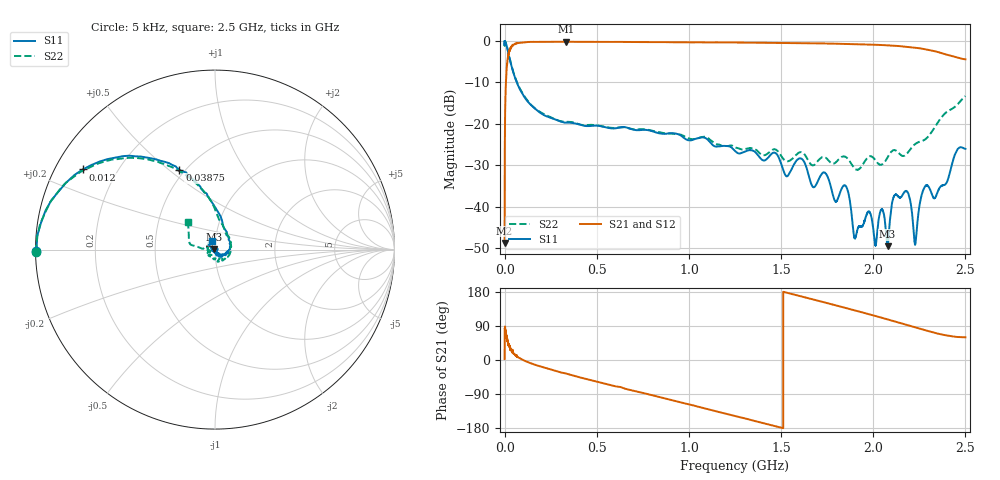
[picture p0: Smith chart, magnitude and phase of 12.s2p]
#  HZ  S  MA  R  50.00
! Rohde & Schwarz Vector Network Analyzer
! Rohde-Schwarz,ZNL6-2Port,1323001206101378,1.50.1.34-21.10.1.104
! Created: UTC 3/3/2025, 4:59:50 AM
! freq[Hz]  mag:S11  ang:S11  mag:S21  ang:S21  mag:S12  ang:S12  mag:S22  ang:S22
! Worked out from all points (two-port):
!   10001 points, 5 kHz to 2.5 GHz, reference 50 ohm
!   highest |S21| = -0.17 dB at 332 MHz (marker M1); lowest = -48.8 dB at 5 kHz (marker M2)
!   |S21| within 3 dB of the highest: 21.47 MHz to 2.389 GHz (2.367 GHz wide, 196 % of centre)
!   lowest |S11| = -49.5 dB at 2.078 GHz (marker M3), VSWR 1.01, Z = 49.7 + j0.0807 ohm
!   |S11| at or under -10 dB: 66.27 MHz to end of sweep
!   |S22| runs from -31.1 to 0.1 dB; largest |S21 - S12| = 0.17
!   S11 on the Smith chart (normalised r, x): 5 kHz: 0.00, -0.00; 12 MHz: 0.08, +0.28; 38.75 MHz: 0.47, +0.54; 2.5 GHz: 0.96, +0.09
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5000  0.9948 -179.6  0.003639 2.5  0.003638 4.6  0.997 -179.3
1.200498e7  0.861 148.7  0.4854 57.6  0.4834 57.3  0.8648 149.9
3.875492e7  0.4868 114.0  0.862 24.1  0.863 24.3  0.4919 115.4
3.320043e8  0.1035 52.3  0.9812 -35.4  0.9811 -35.7  0.106 43.7
4.167542e8  0.09673 37.2  0.9777 -46.9  0.9776 -47.3  0.09698 33.8
8.335033e8  0.07735 -1.2  0.9699 -97.2  0.9725 -97.6  0.07981 -32.3
1.250002e9  0.04715 -34.9  0.9598 -147.8  0.9631 -148.2  0.05201 -95.2
1.608752e9  0.0382 -53.7  0.943 167.9  0.9459 168.1  0.04567 -155.1
1.666752e9  0.01807 -64.8  0.9391 160.7  0.9418 160.9  0.03179 -153.4
1.850251e9  0.01779 -93.7  0.9235 137.3  0.9261 137.6  0.03989 -172.9
1.902001e9  0.004131 20.4  0.9176 130.6  0.9202 130.9  0.02855 -165.8
1.975501e9  0.008707 -127.2  0.9074 120.9  0.9095 121.2  0.04008 178.4
2.013251e9  0.003442 -15.6  0.9006 115.9  0.9029 116.2  0.03607 179.3
2.046501e9  0.00928 75.4  0.8944 111.4  0.896 111.7  0.03228 -172.8
2.077751e9  0.003334 165.9  0.8866 107.1  0.8888 107.4  0.03931 171.8
2.083501e9  0.004286 -152.6  0.885 106.4  0.8873 106.6  0.04136 168.3
2.112251e9  0.01328 -95.5  0.877 102.5  0.8794 102.7  0.04824 158.1
2.177501e9  0.01546 11.4  0.8546 93.3  0.8563 93.5  0.04256 -179.8
2.229001e9  0.003588 -41.1  0.8301 86.1  0.8315 86.3  0.05732 172.5
2.278e9  0.01716 -66.7  0.7988 79.1  0.8 79.4  0.06408 174.9
2.33625e9  0.01285 -116.1  0.7505 71.5  0.7508 71.6  0.09292 171.7
2.5e9  0.04985 110.9  0.6018 59.9  0.6034 59.7  0.2165 134.0
